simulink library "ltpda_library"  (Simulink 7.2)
settings: Solver=ode45  SolverMode=SingleTasking  StartTime=0.0  StopTime=10.0  RelTol=1e-3
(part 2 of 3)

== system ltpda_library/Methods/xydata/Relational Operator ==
  eq : Subsystem  Tag=method xydata  AncestorBlock=libraryBase/function
  ne : Subsystem  Tag=method xydata  AncestorBlock=libraryBase/function

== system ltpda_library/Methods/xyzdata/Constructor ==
  xyzdata : Subsystem  Tag=method xyzdata  AncestorBlock=libraryBase/constructor

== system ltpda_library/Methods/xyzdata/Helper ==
  isprop : Subsystem  Tag=method xyzdata  AncestorBlock=libraryBase/function

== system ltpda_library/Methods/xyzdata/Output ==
  char : Subsystem  Tag=method xyzdata  AncestorBlock=libraryBase/output
  display : Subsystem  Tag=method xyzdata  AncestorBlock=libraryBase/output

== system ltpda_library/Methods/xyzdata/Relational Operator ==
  eq : Subsystem  Tag=method xyzdata  AncestorBlock=libraryBase/function
  ne : Subsystem  Tag=method xyzdata  AncestorBlock=libraryBase/function

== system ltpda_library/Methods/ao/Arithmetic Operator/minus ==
  In1 : Inport  OutDataType=sfix(16)  OutScaling=2^0
  minus : M-S-Function  Tag=minus  FunctionName=ltpdasim
  Out1 : Outport  OutDataType=sfix(16)  OutScaling=2^0
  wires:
  In1/1 -> minus/1
  minus/1 -> Out1/1

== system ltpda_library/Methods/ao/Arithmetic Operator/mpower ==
  In1 : Inport  OutDataType=sfix(16)  OutScaling=2^0
  mpower : M-S-Function  Tag=mpower  FunctionName=ltpdasim
  Out1 : Outport  OutDataType=sfix(16)  OutScaling=2^0
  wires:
  In1/1 -> mpower/1
  mpower/1 -> Out1/1

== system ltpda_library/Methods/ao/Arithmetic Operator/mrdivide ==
  In1 : Inport  OutDataType=sfix(16)  OutScaling=2^0
  mrdivide : M-S-Function  Tag=mrdivide  FunctionName=ltpdasim
  Out1 : Outport  OutDataType=sfix(16)  OutScaling=2^0
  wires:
  In1/1 -> mrdivide/1
  mrdivide/1 -> Out1/1

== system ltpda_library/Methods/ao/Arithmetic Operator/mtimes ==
  In1 : Inport  OutDataType=sfix(16)  OutScaling=2^0
  mtimes : M-S-Function  Tag=mtimes  FunctionName=ltpdasim
  Out1 : Outport  OutDataType=sfix(16)  OutScaling=2^0
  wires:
  In1/1 -> mtimes/1
  mtimes/1 -> Out1/1

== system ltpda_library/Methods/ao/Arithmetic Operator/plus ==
  In1 : Inport  OutDataType=sfix(16)  OutScaling=2^0
  plus : M-S-Function  Tag=plus  FunctionName=ltpdasim
  Out1 : Outport  OutDataType=sfix(16)  OutScaling=2^0
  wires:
  In1/1 -> plus/1
  plus/1 -> Out1/1

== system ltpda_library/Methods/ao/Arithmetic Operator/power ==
  In1 : Inport  OutDataType=sfix(16)  OutScaling=2^0
  power : M-S-Function  Tag=power  FunctionName=ltpdasim
  Out1 : Outport  OutDataType=sfix(16)  OutScaling=2^0
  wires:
  In1/1 -> power/1
  power/1 -> Out1/1

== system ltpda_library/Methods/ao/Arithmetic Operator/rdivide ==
  In1 : Inport  OutDataType=sfix(16)  OutScaling=2^0
  rdivide : M-S-Function  Tag=rdivide  FunctionName=ltpdasim
  Out1 : Outport  OutDataType=sfix(16)  OutScaling=2^0
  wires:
  In1/1 -> rdivide/1
  rdivide/1 -> Out1/1

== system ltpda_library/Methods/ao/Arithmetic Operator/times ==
  In1 : Inport  OutDataType=sfix(16)  OutScaling=2^0
  times : M-S-Function  Tag=times  FunctionName=ltpdasim
  Out1 : Outport  OutDataType=sfix(16)  OutScaling=2^0
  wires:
  In1/1 -> times/1
  times/1 -> Out1/1

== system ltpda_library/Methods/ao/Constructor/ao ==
  Ground : Ground
  ao : M-S-Function  Tag=ao  FunctionName=ltpdasim
  Out1 : Outport  OutDataType=sfix(16)  OutScaling=2^0
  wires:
  Ground/1 -> ao/1
  ao/1 -> Out1/1

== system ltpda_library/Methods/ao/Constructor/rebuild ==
  Ground : Ground
  rebuild : M-S-Function  Tag=rebuild  FunctionName=ltpdasim
  Out1 : Outport  OutDataType=sfix(16)  OutScaling=2^0
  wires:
  Ground/1 -> rebuild/1
  rebuild/1 -> Out1/1

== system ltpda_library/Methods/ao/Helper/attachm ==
  In1 : Inport  OutDataType=sfix(16)  OutScaling=2^0
  attachm : M-S-Function  Tag=attachm  FunctionName=ltpdasim
  Out1 : Outport  OutDataType=sfix(16)  OutScaling=2^0
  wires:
  In1/1 -> attachm/1
  attachm/1 -> Out1/1

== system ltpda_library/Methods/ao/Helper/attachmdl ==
  In1 : Inport  OutDataType=sfix(16)  OutScaling=2^0
  attachmdl : M-S-Function  Tag=attachmdl  FunctionName=ltpdasim
  Out1 : Outport  OutDataType=sfix(16)  OutScaling=2^0
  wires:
  In1/1 -> attachmdl/1
  attachmdl/1 -> Out1/1

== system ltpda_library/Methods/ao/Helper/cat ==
  In1 : Inport  OutDataType=sfix(16)  OutScaling=2^0
  cat : M-S-Function  Tag=cat  FunctionName=ltpdasim
  Out1 : Outport  OutDataType=sfix(16)  OutScaling=2^0
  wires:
  In1/1 -> cat/1
  cat/1 -> Out1/1

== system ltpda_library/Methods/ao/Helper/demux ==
  In1 : Inport  OutDataType=sfix(16)  OutScaling=2^0
  demux : M-S-Function  Tag=demux  FunctionName=ltpdasim
  Out1 : Outport  OutDataType=sfix(16)  OutScaling=2^0
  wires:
  In1/1 -> demux/1
  demux/1 -> Out1/1

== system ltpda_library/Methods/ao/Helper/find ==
  In1 : Inport  OutDataType=sfix(16)  OutScaling=2^0
  find : M-S-Function  Tag=find  FunctionName=ltpdasim
  Out1 : Outport  OutDataType=sfix(16)  OutScaling=2^0
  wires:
  In1/1 -> find/1
  find/1 -> Out1/1

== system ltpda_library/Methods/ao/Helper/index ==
  In1 : Inport  OutDataType=sfix(16)  OutScaling=2^0
  index : M-S-Function  Tag=index  FunctionName=ltpdasim
  Out1 : Outport  OutDataType=sfix(16)  OutScaling=2^0
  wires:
  In1/1 -> index/1
  index/1 -> Out1/1

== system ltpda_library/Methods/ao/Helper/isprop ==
  In1 : Inport  OutDataType=sfix(16)  OutScaling=2^0
  isprop : M-S-Function  Tag=isprop  FunctionName=ltpdasim
  Out1 : Outport  OutDataType=sfix(16)  OutScaling=2^0
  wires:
  In1/1 -> isprop/1
  isprop/1 -> Out1/1

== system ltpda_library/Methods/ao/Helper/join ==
  In1 : Inport  OutDataType=sfix(16)  OutScaling=2^0
  join : M-S-Function  Tag=join  FunctionName=ltpdasim
  Out1 : Outport  OutDataType=sfix(16)  OutScaling=2^0
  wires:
  In1/1 -> join/1
  join/1 -> Out1/1

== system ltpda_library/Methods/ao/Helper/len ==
  In1 : Inport  OutDataType=sfix(16)  OutScaling=2^0
  len : M-S-Function  Tag=len  FunctionName=ltpdasim
  Out1 : Outport  OutDataType=sfix(16)  OutScaling=2^0
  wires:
  In1/1 -> len/1
  len/1 -> Out1/1

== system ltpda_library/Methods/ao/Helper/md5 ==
  In1 : Inport  OutDataType=sfix(16)  OutScaling=2^0
  md5 : M-S-Function  Tag=md5  FunctionName=ltpdasim
  Out1 : Outport  OutDataType=sfix(16)  OutScaling=2^0
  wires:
  In1/1 -> md5/1
  md5/1 -> Out1/1

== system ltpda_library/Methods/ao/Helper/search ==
  In1 : Inport  OutDataType=sfix(16)  OutScaling=2^0
  search : M-S-Function  Tag=search  FunctionName=ltpdasim
  Out1 : Outport  OutDataType=sfix(16)  OutScaling=2^0
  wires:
  In1/1 -> search/1
  search/1 -> Out1/1

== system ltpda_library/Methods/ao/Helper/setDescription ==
  In1 : Inport  OutDataType=sfix(16)  OutScaling=2^0
  setDescription : M-S-Function  Tag=setDescription  FunctionName=ltpdasim
  Out1 : Outport  OutDataType=sfix(16)  OutScaling=2^0
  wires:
  In1/1 -> setDescription/1
  setDescription/1 -> Out1/1

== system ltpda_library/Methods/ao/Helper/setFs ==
  In1 : Inport  OutDataType=sfix(16)  OutScaling=2^0
  setFs : M-S-Function  Tag=setFs  FunctionName=ltpdasim
  Out1 : Outport  OutDataType=sfix(16)  OutScaling=2^0
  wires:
  In1/1 -> setFs/1
  setFs/1 -> Out1/1

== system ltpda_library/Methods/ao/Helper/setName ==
  In1 : Inport  OutDataType=sfix(16)  OutScaling=2^0
  setName : M-S-Function  Tag=setName  FunctionName=ltpdasim
  Out1 : Outport  OutDataType=sfix(16)  OutScaling=2^0
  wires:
  In1/1 -> setName/1
  setName/1 -> Out1/1

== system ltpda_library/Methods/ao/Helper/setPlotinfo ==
  In1 : Inport  OutDataType=sfix(16)  OutScaling=2^0
  setPlotinfo : M-S-Function  Tag=setPlotinfo  FunctionName=ltpdasim
  Out1 : Outport  OutDataType=sfix(16)  OutScaling=2^0
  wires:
  In1/1 -> setPlotinfo/1
  setPlotinfo/1 -> Out1/1

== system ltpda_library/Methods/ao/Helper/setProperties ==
  In1 : Inport  OutDataType=sfix(16)  OutScaling=2^0
  setProperties : M-S-Function  Tag=setProperties  FunctionName=ltpdasim
  Out1 : Outport  OutDataType=sfix(16)  OutScaling=2^0
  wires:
  In1/1 -> setProperties/1
  setProperties/1 -> Out1/1

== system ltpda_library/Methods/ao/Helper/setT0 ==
  In1 : Inport  OutDataType=sfix(16)  OutScaling=2^0
  setT0 : M-S-Function  Tag=setT0  FunctionName=ltpdasim
  Out1 : Outport  OutDataType=sfix(16)  OutScaling=2^0
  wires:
  In1/1 -> setT0/1
  setT0/1 -> Out1/1

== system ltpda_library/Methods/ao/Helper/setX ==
  In1 : Inport  OutDataType=sfix(16)  OutScaling=2^0
  setX : M-S-Function  Tag=setX  FunctionName=ltpdasim
  Out1 : Outport  OutDataType=sfix(16)  OutScaling=2^0
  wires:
  In1/1 -> setX/1
  setX/1 -> Out1/1

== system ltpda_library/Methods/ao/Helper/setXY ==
  In1 : Inport  OutDataType=sfix(16)  OutScaling=2^0
  setXY : M-S-Function  Tag=setXY  FunctionName=ltpdasim
  Out1 : Outport  OutDataType=sfix(16)  OutScaling=2^0
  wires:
  In1/1 -> setXY/1
  setXY/1 -> Out1/1

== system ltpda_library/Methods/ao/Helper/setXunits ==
  In1 : Inport  OutDataType=sfix(16)  OutScaling=2^0
  setXunits : M-S-Function  Tag=setXunits  FunctionName=ltpdasim
  Out1 : Outport  OutDataType=sfix(16)  OutScaling=2^0
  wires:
  In1/1 -> setXunits/1
  setXunits/1 -> Out1/1

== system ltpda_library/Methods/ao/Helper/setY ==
  In1 : Inport  OutDataType=sfix(16)  OutScaling=2^0
  setY : M-S-Function  Tag=setY  FunctionName=ltpdasim
  Out1 : Outport  OutDataType=sfix(16)  OutScaling=2^0
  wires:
  In1/1 -> setY/1
  setY/1 -> Out1/1

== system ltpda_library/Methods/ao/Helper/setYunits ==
  In1 : Inport  OutDataType=sfix(16)  OutScaling=2^0
  setYunits : M-S-Function  Tag=setYunits  FunctionName=ltpdasim
  Out1 : Outport  OutDataType=sfix(16)  OutScaling=2^0
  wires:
  In1/1 -> setYunits/1
  setYunits/1 -> Out1/1

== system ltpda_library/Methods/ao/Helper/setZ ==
  In1 : Inport  OutDataType=sfix(16)  OutScaling=2^0
  setZ : M-S-Function  Tag=setZ  FunctionName=ltpdasim
  Out1 : Outport  OutDataType=sfix(16)  OutScaling=2^0
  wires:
  In1/1 -> setZ/1
  setZ/1 -> Out1/1

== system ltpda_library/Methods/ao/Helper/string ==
  In1 : Inport  OutDataType=sfix(16)  OutScaling=2^0
  string : M-S-Function  Tag=string  FunctionName=ltpdasim
  Out1 : Outport  OutDataType=sfix(16)  OutScaling=2^0
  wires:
  In1/1 -> string/1
  string/1 -> Out1/1

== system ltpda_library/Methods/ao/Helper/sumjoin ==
  In1 : Inport  OutDataType=sfix(16)  OutScaling=2^0
  sumjoin : M-S-Function  Tag=sumjoin  FunctionName=ltpdasim
  Out1 : Outport  OutDataType=sfix(16)  OutScaling=2^0
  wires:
  In1/1 -> sumjoin/1
  sumjoin/1 -> Out1/1

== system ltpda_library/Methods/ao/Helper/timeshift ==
  In1 : Inport  OutDataType=sfix(16)  OutScaling=2^0
  timeshift : M-S-Function  Tag=timeshift  FunctionName=ltpdasim
  Out1 : Outport  OutDataType=sfix(16)  OutScaling=2^0
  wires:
  In1/1 -> timeshift/1
  timeshift/1 -> Out1/1

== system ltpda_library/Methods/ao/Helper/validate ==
  In1 : Inport  OutDataType=sfix(16)  OutScaling=2^0
  validate : M-S-Function  Tag=validate  FunctionName=ltpdasim
  Out1 : Outport  OutDataType=sfix(16)  OutScaling=2^0
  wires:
  In1/1 -> validate/1
  validate/1 -> Out1/1

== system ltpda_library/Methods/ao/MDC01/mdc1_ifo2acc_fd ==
  In1 : Inport  OutDataType=sfix(16)  OutScaling=2^0
  mdc1_ifo2acc_fd : M-S-Function  Tag=mdc1_ifo2acc_fd  FunctionName=ltpdasim
  Out1 : Outport  OutDataType=sfix(16)  OutScaling=2^0
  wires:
  In1/1 -> mdc1_ifo2acc_fd/1
  mdc1_ifo2acc_fd/1 -> Out1/1

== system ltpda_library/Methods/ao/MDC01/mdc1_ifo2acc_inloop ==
  In1 : Inport  OutDataType=sfix(16)  OutScaling=2^0
  mdc1_ifo2acc_inloop : M-S-Function  Tag=mdc1_ifo2acc_inloop  FunctionName=ltpdasim
  Out1 : Outport  OutDataType=sfix(16)  OutScaling=2^0
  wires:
  In1/1 -> mdc1_ifo2acc_inloop/1
  mdc1_ifo2acc_inloop/1 -> Out1/1

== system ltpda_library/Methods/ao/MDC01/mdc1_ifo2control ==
  In1 : Inport  OutDataType=sfix(16)  OutScaling=2^0
  mdc1_ifo2control : M-S-Function  Tag=mdc1_ifo2control  FunctionName=ltpdasim
  Out1 : Outport  OutDataType=sfix(16)  OutScaling=2^0
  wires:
  In1/1 -> mdc1_ifo2control/1
  mdc1_ifo2control/1 -> Out1/1

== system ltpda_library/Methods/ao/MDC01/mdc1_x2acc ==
  In1 : Inport  OutDataType=sfix(16)  OutScaling=2^0
  mdc1_x2acc : M-S-Function  Tag=mdc1_x2acc  FunctionName=ltpdasim
  Out1 : Outport  OutDataType=sfix(16)  OutScaling=2^0
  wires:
  In1/1 -> mdc1_x2acc/1
  mdc1_x2acc/1 -> Out1/1

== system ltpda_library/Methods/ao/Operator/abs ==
  In1 : Inport  OutDataType=sfix(16)  OutScaling=2^0
  abs : M-S-Function  Tag=abs  FunctionName=ltpdasim
  Out1 : Outport  OutDataType=sfix(16)  OutScaling=2^0
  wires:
  In1/1 -> abs/1
  abs/1 -> Out1/1

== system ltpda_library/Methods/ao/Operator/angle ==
  In1 : Inport  OutDataType=sfix(16)  OutScaling=2^0
  angle : M-S-Function  Tag=angle  FunctionName=ltpdasim
  Out1 : Outport  OutDataType=sfix(16)  OutScaling=2^0
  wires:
  In1/1 -> angle/1
  angle/1 -> Out1/1

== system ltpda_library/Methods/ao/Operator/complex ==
  In1 : Inport  OutDataType=sfix(16)  OutScaling=2^0
  complex : M-S-Function  Tag=complex  FunctionName=ltpdasim
  Out1 : Outport  OutDataType=sfix(16)  OutScaling=2^0
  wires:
  In1/1 -> complex/1
  complex/1 -> Out1/1

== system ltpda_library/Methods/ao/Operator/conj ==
  In1 : Inport  OutDataType=sfix(16)  OutScaling=2^0
  conj : M-S-Function  Tag=conj  FunctionName=ltpdasim
  Out1 : Outport  OutDataType=sfix(16)  OutScaling=2^0
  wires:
  In1/1 -> conj/1
  conj/1 -> Out1/1

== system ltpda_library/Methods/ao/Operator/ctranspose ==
  In1 : Inport  OutDataType=sfix(16)  OutScaling=2^0
  ctranspose : M-S-Function  Tag=ctranspose  FunctionName=ltpdasim
  Out1 : Outport  OutDataType=sfix(16)  OutScaling=2^0
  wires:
  In1/1 -> ctranspose/1
  ctranspose/1 -> Out1/1

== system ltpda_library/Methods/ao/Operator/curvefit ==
  In1 : Inport  OutDataType=sfix(16)  OutScaling=2^0
  curvefit : M-S-Function  Tag=curvefit  FunctionName=ltpdasim
  Out1 : Outport  OutDataType=sfix(16)  OutScaling=2^0
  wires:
  In1/1 -> curvefit/1
  curvefit/1 -> Out1/1

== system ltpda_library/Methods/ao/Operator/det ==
  In1 : Inport  OutDataType=sfix(16)  OutScaling=2^0
  det : M-S-Function  Tag=det  FunctionName=ltpdasim
  Out1 : Outport  OutDataType=sfix(16)  OutScaling=2^0
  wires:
  In1/1 -> det/1
  det/1 -> Out1/1

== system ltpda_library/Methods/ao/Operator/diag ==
  In1 : Inport  OutDataType=sfix(16)  OutScaling=2^0
  diag : M-S-Function  Tag=diag  FunctionName=ltpdasim
  Out1 : Outport  OutDataType=sfix(16)  OutScaling=2^0
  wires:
  In1/1 -> diag/1
  diag/1 -> Out1/1

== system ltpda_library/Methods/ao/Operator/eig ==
  In1 : Inport  OutDataType=sfix(16)  OutScaling=2^0
  eig : M-S-Function  Tag=eig  FunctionName=ltpdasim
  Out1 : Outport  OutDataType=sfix(16)  OutScaling=2^0
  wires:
  In1/1 -> eig/1
  eig/1 -> Out1/1

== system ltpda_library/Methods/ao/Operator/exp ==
  In1 : Inport  OutDataType=sfix(16)  OutScaling=2^0
  exp : M-S-Function  Tag=exp  FunctionName=ltpdasim
  Out1 : Outport  OutDataType=sfix(16)  OutScaling=2^0
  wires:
  In1/1 -> exp/1
  exp/1 -> Out1/1

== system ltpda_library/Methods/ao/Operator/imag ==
  In1 : Inport  OutDataType=sfix(16)  OutScaling=2^0
  imag : M-S-Function  Tag=imag  FunctionName=ltpdasim
  Out1 : Outport  OutDataType=sfix(16)  OutScaling=2^0
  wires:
  In1/1 -> imag/1
  imag/1 -> Out1/1

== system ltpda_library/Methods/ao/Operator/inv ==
  In1 : Inport  OutDataType=sfix(16)  OutScaling=2^0
  inv : M-S-Function  Tag=inv  FunctionName=ltpdasim
  Out1 : Outport  OutDataType=sfix(16)  OutScaling=2^0
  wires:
  In1/1 -> inv/1
  inv/1 -> Out1/1

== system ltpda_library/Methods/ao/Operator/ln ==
  In1 : Inport  OutDataType=sfix(16)  OutScaling=2^0
  ln : M-S-Function  Tag=ln  FunctionName=ltpdasim
  Out1 : Outport  OutDataType=sfix(16)  OutScaling=2^0
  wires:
  In1/1 -> ln/1
  ln/1 -> Out1/1

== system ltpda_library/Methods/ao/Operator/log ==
  In1 : Inport  OutDataType=sfix(16)  OutScaling=2^0
  log : M-S-Function  Tag=log  FunctionName=ltpdasim
  Out1 : Outport  OutDataType=sfix(16)  OutScaling=2^0
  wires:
  In1/1 -> log/1
  log/1 -> Out1/1

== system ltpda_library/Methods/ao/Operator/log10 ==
  In1 : Inport  OutDataType=sfix(16)  OutScaling=2^0
  log10 : M-S-Function  Tag=log10  FunctionName=ltpdasim
  Out1 : Outport  OutDataType=sfix(16)  OutScaling=2^0
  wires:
  In1/1 -> log10/1
  log10/1 -> Out1/1

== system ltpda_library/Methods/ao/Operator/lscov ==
  In1 : Inport  OutDataType=sfix(16)  OutScaling=2^0
  lscov : M-S-Function  Tag=lscov  FunctionName=ltpdasim
  Out1 : Outport  OutDataType=sfix(16)  OutScaling=2^0
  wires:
  In1/1 -> lscov/1
  lscov/1 -> Out1/1

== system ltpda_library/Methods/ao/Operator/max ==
  In1 : Inport  OutDataType=sfix(16)  OutScaling=2^0
  max : M-S-Function  Tag=max  FunctionName=ltpdasim
  Out1 : Outport  OutDataType=sfix(16)  OutScaling=2^0
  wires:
  In1/1 -> max/1
  max/1 -> Out1/1

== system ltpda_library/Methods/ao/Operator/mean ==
  In1 : Inport  OutDataType=sfix(16)  OutScaling=2^0
  mean : M-S-Function  Tag=mean  FunctionName=ltpdasim
  Out1 : Outport  OutDataType=sfix(16)  OutScaling=2^0
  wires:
  In1/1 -> mean/1
  mean/1 -> Out1/1

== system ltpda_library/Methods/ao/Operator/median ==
  In1 : Inport  OutDataType=sfix(16)  OutScaling=2^0
  median : M-S-Function  Tag=median  FunctionName=ltpdasim
  Out1 : Outport  OutDataType=sfix(16)  OutScaling=2^0
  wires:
  In1/1 -> median/1
  median/1 -> Out1/1

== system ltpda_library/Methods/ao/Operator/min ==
  In1 : Inport  OutDataType=sfix(16)  OutScaling=2^0
  min : M-S-Function  Tag=min  FunctionName=ltpdasim
  Out1 : Outport  OutDataType=sfix(16)  OutScaling=2^0
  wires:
  In1/1 -> min/1
  min/1 -> Out1/1

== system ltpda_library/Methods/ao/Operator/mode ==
  In1 : Inport  OutDataType=sfix(16)  OutScaling=2^0
  mode : M-S-Function  Tag=mode  FunctionName=ltpdasim
  Out1 : Outport  OutDataType=sfix(16)  OutScaling=2^0
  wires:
  In1/1 -> mode/1
  mode/1 -> Out1/1

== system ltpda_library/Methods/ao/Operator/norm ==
  In1 : Inport  OutDataType=sfix(16)  OutScaling=2^0
  norm : M-S-Function  Tag=norm  FunctionName=ltpdasim
  Out1 : Outport  OutDataType=sfix(16)  OutScaling=2^0
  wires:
  In1/1 -> norm/1
  norm/1 -> Out1/1

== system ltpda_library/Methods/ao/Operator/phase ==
  In1 : Inport  OutDataType=sfix(16)  OutScaling=2^0
  phase : M-S-Function  Tag=phase  FunctionName=ltpdasim
  Out1 : Outport  OutDataType=sfix(16)  OutScaling=2^0
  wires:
  In1/1 -> phase/1
  phase/1 -> Out1/1

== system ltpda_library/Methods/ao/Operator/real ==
  In1 : Inport  OutDataType=sfix(16)  OutScaling=2^0
  real : M-S-Function  Tag=real  FunctionName=ltpdasim
  Out1 : Outport  OutDataType=sfix(16)  OutScaling=2^0
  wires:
  In1/1 -> real/1
  real/1 -> Out1/1

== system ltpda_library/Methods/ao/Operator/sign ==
  In1 : Inport  OutDataType=sfix(16)  OutScaling=2^0
  sign : M-S-Function  Tag=sign  FunctionName=ltpdasim
  Out1 : Outport  OutDataType=sfix(16)  OutScaling=2^0
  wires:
  In1/1 -> sign/1
  sign/1 -> Out1/1

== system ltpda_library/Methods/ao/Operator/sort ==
  In1 : Inport  OutDataType=sfix(16)  OutScaling=2^0
  sort : M-S-Function  Tag=sort  FunctionName=ltpdasim
  Out1 : Outport  OutDataType=sfix(16)  OutScaling=2^0
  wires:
  In1/1 -> sort/1
  sort/1 -> Out1/1

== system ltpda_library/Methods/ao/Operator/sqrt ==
  In1 : Inport  OutDataType=sfix(16)  OutScaling=2^0
  sqrt : M-S-Function  Tag=sqrt  FunctionName=ltpdasim
  Out1 : Outport  OutDataType=sfix(16)  OutScaling=2^0
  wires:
  In1/1 -> sqrt/1
  sqrt/1 -> Out1/1

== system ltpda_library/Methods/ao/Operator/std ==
  In1 : Inport  OutDataType=sfix(16)  OutScaling=2^0
  std : M-S-Function  Tag=std  FunctionName=ltpdasim
  Out1 : Outport  OutDataType=sfix(16)  OutScaling=2^0
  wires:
  In1/1 -> std/1
  std/1 -> Out1/1

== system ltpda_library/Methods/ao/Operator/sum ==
  In1 : Inport  OutDataType=sfix(16)  OutScaling=2^0
  sum : M-S-Function  Tag=sum  FunctionName=ltpdasim
  Out1 : Outport  OutDataType=sfix(16)  OutScaling=2^0
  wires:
  In1/1 -> sum/1
  sum/1 -> Out1/1

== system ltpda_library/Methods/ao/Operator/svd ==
  In1 : Inport  OutDataType=sfix(16)  OutScaling=2^0
  svd : M-S-Function  Tag=svd  FunctionName=ltpdasim
  Out1 : Outport  OutDataType=sfix(16)  OutScaling=2^0
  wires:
  In1/1 -> svd/1
  svd/1 -> Out1/1

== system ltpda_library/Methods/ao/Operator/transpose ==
  In1 : Inport  OutDataType=sfix(16)  OutScaling=2^0
  transpose : M-S-Function  Tag=transpose  FunctionName=ltpdasim
  Out1 : Outport  OutDataType=sfix(16)  OutScaling=2^0
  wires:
  In1/1 -> transpose/1
  transpose/1 -> Out1/1

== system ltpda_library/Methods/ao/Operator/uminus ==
  In1 : Inport  OutDataType=sfix(16)  OutScaling=2^0
  uminus : M-S-Function  Tag=uminus  FunctionName=ltpdasim
  Out1 : Outport  OutDataType=sfix(16)  OutScaling=2^0
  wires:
  In1/1 -> uminus/1
  uminus/1 -> Out1/1

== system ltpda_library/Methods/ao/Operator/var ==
  In1 : Inport  OutDataType=sfix(16)  OutScaling=2^0
  var : M-S-Function  Tag=var  FunctionName=ltpdasim
  Out1 : Outport  OutDataType=sfix(16)  OutScaling=2^0
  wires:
  In1/1 -> var/1
  var/1 -> Out1/1

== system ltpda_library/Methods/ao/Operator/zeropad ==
  In1 : Inport  OutDataType=sfix(16)  OutScaling=2^0
  zeropad : M-S-Function  Tag=zeropad  FunctionName=ltpdasim
  Out1 : Outport  OutDataType=sfix(16)  OutScaling=2^0
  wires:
  In1/1 -> zeropad/1
  zeropad/1 -> Out1/1

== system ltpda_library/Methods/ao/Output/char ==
  In1 : Inport  OutDataType=sfix(16)  OutScaling=2^0
  Terminator : Terminator
  char : M-S-Function  Tag=char  FunctionName=ltpdasim
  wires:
  char/1 -> Terminator/1
  In1/1 -> char/1

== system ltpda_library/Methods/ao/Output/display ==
  In1 : Inport  OutDataType=sfix(16)  OutScaling=2^0
  Terminator : Terminator
  display : M-S-Function  Tag=display  FunctionName=ltpdasim
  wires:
  display/1 -> Terminator/1
  In1/1 -> display/1

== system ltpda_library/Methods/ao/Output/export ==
  In1 : Inport  OutDataType=sfix(16)  OutScaling=2^0
  Terminator : Terminator
  export : M-S-Function  Tag=export  FunctionName=ltpdasim
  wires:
  export/1 -> Terminator/1
  In1/1 -> export/1

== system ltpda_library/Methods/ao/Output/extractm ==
  In1 : Inport  OutDataType=sfix(16)  OutScaling=2^0
  Terminator : Terminator
  extractm : M-S-Function  Tag=extractm  FunctionName=ltpdasim
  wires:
  extractm/1 -> Terminator/1
  In1/1 -> extractm/1

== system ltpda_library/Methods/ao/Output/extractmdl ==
  In1 : Inport  OutDataType=sfix(16)  OutScaling=2^0
  Terminator : Terminator
  extractmdl : M-S-Function  Tag=extractmdl  FunctionName=ltpdasim
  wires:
  extractmdl/1 -> Terminator/1
  In1/1 -> extractmdl/1

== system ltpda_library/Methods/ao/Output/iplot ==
  In1 : Inport  OutDataType=sfix(16)  OutScaling=2^0
  Terminator : Terminator
  iplot : M-S-Function  Tag=iplot  FunctionName=ltpdasim
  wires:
  iplot/1 -> Terminator/1
  In1/1 -> iplot/1

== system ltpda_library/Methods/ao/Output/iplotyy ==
  In1 : Inport  OutDataType=sfix(16)  OutScaling=2^0
  Terminator : Terminator
  iplotyy : M-S-Function  Tag=iplotyy  FunctionName=ltpdasim
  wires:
  iplotyy/1 -> Terminator/1
  In1/1 -> iplotyy/1

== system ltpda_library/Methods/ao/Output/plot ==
  In1 : Inport  OutDataType=sfix(16)  OutScaling=2^0
  Terminator : Terminator
  plot : M-S-Function  Tag=plot  FunctionName=ltpdasim
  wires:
  plot/1 -> Terminator/1
  In1/1 -> plot/1

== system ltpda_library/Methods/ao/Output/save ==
  In1 : Inport  OutDataType=sfix(16)  OutScaling=2^0
  Terminator : Terminator
  save : M-S-Function  Tag=save  FunctionName=ltpdasim
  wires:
  save/1 -> Terminator/1
  In1/1 -> save/1

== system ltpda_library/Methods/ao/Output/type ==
  In1 : Inport  OutDataType=sfix(16)  OutScaling=2^0
  Terminator : Terminator
  type : M-S-Function  Tag=type  FunctionName=ltpdasim
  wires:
  type/1 -> Terminator/1
  In1/1 -> type/1

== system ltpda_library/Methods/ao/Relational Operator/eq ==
  In1 : Inport  OutDataType=sfix(16)  OutScaling=2^0
  eq : M-S-Function  Tag=eq  FunctionName=ltpdasim
  Out1 : Outport  OutDataType=sfix(16)  OutScaling=2^0
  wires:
  In1/1 -> eq/1
  eq/1 -> Out1/1

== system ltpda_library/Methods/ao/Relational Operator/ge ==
  In1 : Inport  OutDataType=sfix(16)  OutScaling=2^0
  ge : M-S-Function  Tag=ge  FunctionName=ltpdasim
  Out1 : Outport  OutDataType=sfix(16)  OutScaling=2^0
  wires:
  In1/1 -> ge/1
  ge/1 -> Out1/1

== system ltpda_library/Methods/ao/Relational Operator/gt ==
  In1 : Inport  OutDataType=sfix(16)  OutScaling=2^0
  gt : M-S-Function  Tag=gt  FunctionName=ltpdasim
  Out1 : Outport  OutDataType=sfix(16)  OutScaling=2^0
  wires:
  In1/1 -> gt/1
  gt/1 -> Out1/1

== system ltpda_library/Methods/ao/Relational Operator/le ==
  In1 : Inport  OutDataType=sfix(16)  OutScaling=2^0
  le : M-S-Function  Tag=le  FunctionName=ltpdasim
  Out1 : Outport  OutDataType=sfix(16)  OutScaling=2^0
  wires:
  In1/1 -> le/1
  le/1 -> Out1/1

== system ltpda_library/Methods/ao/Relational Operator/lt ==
  In1 : Inport  OutDataType=sfix(16)  OutScaling=2^0
  lt : M-S-Function  Tag=lt  FunctionName=ltpdasim
  Out1 : Outport  OutDataType=sfix(16)  OutScaling=2^0
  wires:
  In1/1 -> lt/1
  lt/1 -> Out1/1

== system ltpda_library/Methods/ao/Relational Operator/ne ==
  In1 : Inport  OutDataType=sfix(16)  OutScaling=2^0
  ne : M-S-Function  Tag=ne  FunctionName=ltpdasim
  Out1 : Outport  OutDataType=sfix(16)  OutScaling=2^0
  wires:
  In1/1 -> ne/1
  ne/1 -> Out1/1

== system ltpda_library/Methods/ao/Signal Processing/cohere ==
  In1 : Inport  OutDataType=sfix(16)  OutScaling=2^0
  cohere : M-S-Function  Tag=cohere  FunctionName=ltpdasim
  Out1 : Outport  OutDataType=sfix(16)  OutScaling=2^0
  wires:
  In1/1 -> cohere/1
  cohere/1 -> Out1/1

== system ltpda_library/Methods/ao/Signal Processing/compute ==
  In1 : Inport  OutDataType=sfix(16)  OutScaling=2^0
  compute : M-S-Function  Tag=compute  FunctionName=ltpdasim
  Out1 : Outport  OutDataType=sfix(16)  OutScaling=2^0
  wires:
  In1/1 -> compute/1
  compute/1 -> Out1/1

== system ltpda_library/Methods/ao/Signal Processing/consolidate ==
  In1 : Inport  OutDataType=sfix(16)  OutScaling=2^0
  consolidate : M-S-Function  Tag=consolidate  FunctionName=ltpdasim
  Out1 : Outport  OutDataType=sfix(16)  OutScaling=2^0
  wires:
  In1/1 -> consolidate/1
  consolidate/1 -> Out1/1

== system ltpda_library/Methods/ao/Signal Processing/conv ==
  In1 : Inport  OutDataType=sfix(16)  OutScaling=2^0
  conv : M-S-Function  Tag=conv  FunctionName=ltpdasim
  Out1 : Outport  OutDataType=sfix(16)  OutScaling=2^0
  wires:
  In1/1 -> conv/1
  conv/1 -> Out1/1

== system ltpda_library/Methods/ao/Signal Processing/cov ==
  In1 : Inport  OutDataType=sfix(16)  OutScaling=2^0
  cov : M-S-Function  Tag=cov  FunctionName=ltpdasim
  Out1 : Outport  OutDataType=sfix(16)  OutScaling=2^0
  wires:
  In1/1 -> cov/1
  cov/1 -> Out1/1

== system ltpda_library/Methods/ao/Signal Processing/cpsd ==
  In1 : Inport  OutDataType=sfix(16)  OutScaling=2^0
  cpsd : M-S-Function  Tag=cpsd  FunctionName=ltpdasim
  Out1 : Outport  OutDataType=sfix(16)  OutScaling=2^0
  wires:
  In1/1 -> cpsd/1
  cpsd/1 -> Out1/1

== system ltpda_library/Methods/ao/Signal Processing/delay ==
  In1 : Inport  OutDataType=sfix(16)  OutScaling=2^0
  delay : M-S-Function  Tag=delay  FunctionName=ltpdasim
  Out1 : Outport  OutDataType=sfix(16)  OutScaling=2^0
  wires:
  In1/1 -> delay/1
  delay/1 -> Out1/1

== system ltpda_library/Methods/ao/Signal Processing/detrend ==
  In1 : Inport  OutDataType=sfix(16)  OutScaling=2^0
  detrend : M-S-Function  Tag=detrend  FunctionName=ltpdasim
  Out1 : Outport  OutDataType=sfix(16)  OutScaling=2^0
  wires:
  In1/1 -> detrend/1
  detrend/1 -> Out1/1

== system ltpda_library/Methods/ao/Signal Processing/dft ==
  In1 : Inport  OutDataType=sfix(16)  OutScaling=2^0
  dft : M-S-Function  Tag=dft  FunctionName=ltpdasim
  Out1 : Outport  OutDataType=sfix(16)  OutScaling=2^0
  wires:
  In1/1 -> dft/1
  dft/1 -> Out1/1

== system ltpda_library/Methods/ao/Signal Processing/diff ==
  In1 : Inport  OutDataType=sfix(16)  OutScaling=2^0
  diff : M-S-Function  Tag=diff  FunctionName=ltpdasim
  Out1 : Outport  OutDataType=sfix(16)  OutScaling=2^0
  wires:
  In1/1 -> diff/1
  diff/1 -> Out1/1

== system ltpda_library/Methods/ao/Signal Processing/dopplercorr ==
  In1 : Inport  OutDataType=sfix(16)  OutScaling=2^0
  dopplercorr : M-S-Function  Tag=dopplercorr  FunctionName=ltpdasim
  Out1 : Outport  OutDataType=sfix(16)  OutScaling=2^0
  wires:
  In1/1 -> dopplercorr/1
  dopplercorr/1 -> Out1/1

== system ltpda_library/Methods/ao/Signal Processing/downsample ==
  In1 : Inport  OutDataType=sfix(16)  OutScaling=2^0
  downsample : M-S-Function  Tag=downsample  FunctionName=ltpdasim
  Out1 : Outport  OutDataType=sfix(16)  OutScaling=2^0
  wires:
  In1/1 -> downsample/1
  downsample/1 -> Out1/1

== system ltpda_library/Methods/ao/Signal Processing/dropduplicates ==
  In1 : Inport  OutDataType=sfix(16)  OutScaling=2^0
  dropduplicates : M-S-Function  Tag=dropduplicates  FunctionName=ltpdasim
  Out1 : Outport  OutDataType=sfix(16)  OutScaling=2^0
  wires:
  In1/1 -> dropduplicates/1
  dropduplicates/1 -> Out1/1

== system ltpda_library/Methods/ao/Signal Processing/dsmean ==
  In1 : Inport  OutDataType=sfix(16)  OutScaling=2^0
  dsmean : M-S-Function  Tag=dsmean  FunctionName=ltpdasim
  Out1 : Outport  OutDataType=sfix(16)  OutScaling=2^0
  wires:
  In1/1 -> dsmean/1
  dsmean/1 -> Out1/1

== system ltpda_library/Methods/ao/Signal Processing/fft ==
  In1 : Inport  OutDataType=sfix(16)  OutScaling=2^0
  fft : M-S-Function  Tag=fft  FunctionName=ltpdasim
  Out1 : Outport  OutDataType=sfix(16)  OutScaling=2^0
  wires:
  In1/1 -> fft/1
  fft/1 -> Out1/1

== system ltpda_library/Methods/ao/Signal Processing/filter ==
  In1 : Inport  OutDataType=sfix(16)  OutScaling=2^0
  filter : M-S-Function  Tag=filter  FunctionName=ltpdasim
  Out1 : Outport  OutDataType=sfix(16)  OutScaling=2^0
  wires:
  In1/1 -> filter/1
  filter/1 -> Out1/1

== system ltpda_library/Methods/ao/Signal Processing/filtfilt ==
  In1 : Inport  OutDataType=sfix(16)  OutScaling=2^0
  filtfilt : M-S-Function  Tag=filtfilt  FunctionName=ltpdasim
  Out1 : Outport  OutDataType=sfix(16)  OutScaling=2^0
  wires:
  In1/1 -> filtfilt/1
  filtfilt/1 -> Out1/1

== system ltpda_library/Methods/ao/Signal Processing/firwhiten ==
  In1 : Inport  OutDataType=sfix(16)  OutScaling=2^0
  firwhiten : M-S-Function  Tag=firwhiten  FunctionName=ltpdasim
  Out1 : Outport  OutDataType=sfix(16)  OutScaling=2^0
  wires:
  In1/1 -> firwhiten/1
  firwhiten/1 -> Out1/1

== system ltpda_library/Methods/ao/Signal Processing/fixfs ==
  In1 : Inport  OutDataType=sfix(16)  OutScaling=2^0
  fixfs : M-S-Function  Tag=fixfs  FunctionName=ltpdasim
  Out1 : Outport  OutDataType=sfix(16)  OutScaling=2^0
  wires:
  In1/1 -> fixfs/1
  fixfs/1 -> Out1/1

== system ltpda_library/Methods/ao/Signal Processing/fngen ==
  In1 : Inport  OutDataType=sfix(16)  OutScaling=2^0
  fngen : M-S-Function  Tag=fngen  FunctionName=ltpdasim
  Out1 : Outport  OutDataType=sfix(16)  OutScaling=2^0
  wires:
  In1/1 -> fngen/1
  fngen/1 -> Out1/1

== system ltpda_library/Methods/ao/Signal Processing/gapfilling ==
  In1 : Inport  OutDataType=sfix(16)  OutScaling=2^0
  gapfilling : M-S-Function  Tag=gapfilling  FunctionName=ltpdasim
  Out1 : Outport  OutDataType=sfix(16)  OutScaling=2^0
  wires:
  In1/1 -> gapfilling/1
  gapfilling/1 -> Out1/1

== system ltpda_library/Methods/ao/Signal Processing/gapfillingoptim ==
  In1 : Inport  OutDataType=sfix(16)  OutScaling=2^0
  gapfillingoptim : M-S-Function  Tag=gapfillingoptim  FunctionName=ltpdasim
  Out1 : Outport  OutDataType=sfix(16)  OutScaling=2^0
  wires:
  In1/1 -> gapfillingoptim/1
  gapfillingoptim/1 -> Out1/1

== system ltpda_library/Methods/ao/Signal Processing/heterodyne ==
  In1 : Inport  OutDataType=sfix(16)  OutScaling=2^0
  heterodyne : M-S-Function  Tag=heterodyne  FunctionName=ltpdasim
  Out1 : Outport  OutDataType=sfix(16)  OutScaling=2^0
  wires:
  In1/1 -> heterodyne/1
  heterodyne/1 -> Out1/1

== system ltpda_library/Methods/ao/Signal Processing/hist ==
  In1 : Inport  OutDataType=sfix(16)  OutScaling=2^0
  hist : M-S-Function  Tag=hist  FunctionName=ltpdasim
  Out1 : Outport  OutDataType=sfix(16)  OutScaling=2^0
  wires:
  In1/1 -> hist/1
  hist/1 -> Out1/1

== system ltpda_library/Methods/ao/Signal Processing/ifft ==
  In1 : Inport  OutDataType=sfix(16)  OutScaling=2^0
  ifft : M-S-Function  Tag=ifft  FunctionName=ltpdasim
  Out1 : Outport  OutDataType=sfix(16)  OutScaling=2^0
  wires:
  In1/1 -> ifft/1
  ifft/1 -> Out1/1

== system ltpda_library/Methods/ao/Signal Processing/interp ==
  In1 : Inport  OutDataType=sfix(16)  OutScaling=2^0
  interp : M-S-Function  Tag=interp  FunctionName=ltpdasim
  Out1 : Outport  OutDataType=sfix(16)  OutScaling=2^0
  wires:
  In1/1 -> interp/1
  interp/1 -> Out1/1

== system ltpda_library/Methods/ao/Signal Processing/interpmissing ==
  In1 : Inport  OutDataType=sfix(16)  OutScaling=2^0
  interpmissing : M-S-Function  Tag=interpmissing  FunctionName=ltpdasim
  Out1 : Outport  OutDataType=sfix(16)  OutScaling=2^0
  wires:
  In1/1 -> interpmissing/1
  interpmissing/1 -> Out1/1

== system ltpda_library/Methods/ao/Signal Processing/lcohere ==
  In1 : Inport  OutDataType=sfix(16)  OutScaling=2^0
  lcohere : M-S-Function  Tag=lcohere  FunctionName=ltpdasim
  Out1 : Outport  OutDataType=sfix(16)  OutScaling=2^0
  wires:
  In1/1 -> lcohere/1
  lcohere/1 -> Out1/1

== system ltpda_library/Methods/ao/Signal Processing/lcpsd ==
  In1 : Inport  OutDataType=sfix(16)  OutScaling=2^0
  lcpsd : M-S-Function  Tag=lcpsd  FunctionName=ltpdasim
  Out1 : Outport  OutDataType=sfix(16)  OutScaling=2^0
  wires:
  In1/1 -> lcpsd/1
  lcpsd/1 -> Out1/1

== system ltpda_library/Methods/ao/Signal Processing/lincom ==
  In1 : Inport  OutDataType=sfix(16)  OutScaling=2^0
  lincom : M-S-Function  Tag=lincom  FunctionName=ltpdasim
  Out1 : Outport  OutDataType=sfix(16)  OutScaling=2^0
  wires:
  In1/1 -> lincom/1
  lincom/1 -> Out1/1

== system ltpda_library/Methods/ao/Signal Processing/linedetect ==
  In1 : Inport  OutDataType=sfix(16)  OutScaling=2^0
  linedetect : M-S-Function  Tag=linedetect  FunctionName=ltpdasim
  Out1 : Outport  OutDataType=sfix(16)  OutScaling=2^0
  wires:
  In1/1 -> linedetect/1
  linedetect/1 -> Out1/1

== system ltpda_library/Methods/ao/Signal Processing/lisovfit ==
  In1 : Inport  OutDataType=sfix(16)  OutScaling=2^0
  lisovfit : M-S-Function  Tag=lisovfit  FunctionName=ltpdasim
  Out1 : Outport  OutDataType=sfix(16)  OutScaling=2^0
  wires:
  In1/1 -> lisovfit/1
  lisovfit/1 -> Out1/1

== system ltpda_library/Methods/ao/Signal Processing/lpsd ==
  In1 : Inport  OutDataType=sfix(16)  OutScaling=2^0
  lpsd : M-S-Function  Tag=lpsd  FunctionName=ltpdasim
  Out1 : Outport  OutDataType=sfix(16)  OutScaling=2^0
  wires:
  In1/1 -> lpsd/1
  lpsd/1 -> Out1/1

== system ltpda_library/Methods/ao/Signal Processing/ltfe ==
  In1 : Inport  OutDataType=sfix(16)  OutScaling=2^0
  ltfe : M-S-Function  Tag=ltfe  FunctionName=ltpdasim
  Out1 : Outport  OutDataType=sfix(16)  OutScaling=2^0
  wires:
  In1/1 -> ltfe/1
  ltfe/1 -> Out1/1

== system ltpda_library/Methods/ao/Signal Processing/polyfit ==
  In1 : Inport  OutDataType=sfix(16)  OutScaling=2^0
  polyfit : M-S-Function  Tag=polyfit  FunctionName=ltpdasim
  Out1 : Outport  OutDataType=sfix(16)  OutScaling=2^0
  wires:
  In1/1 -> polyfit/1
  polyfit/1 -> Out1/1

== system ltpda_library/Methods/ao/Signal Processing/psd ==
  In1 : Inport  OutDataType=sfix(16)  OutScaling=2^0
  psd : M-S-Function  Tag=psd  FunctionName=ltpdasim
  Out1 : Outport  OutDataType=sfix(16)  OutScaling=2^0
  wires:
  In1/1 -> psd/1
  psd/1 -> Out1/1

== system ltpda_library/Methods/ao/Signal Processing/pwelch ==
  In1 : Inport  OutDataType=sfix(16)  OutScaling=2^0
  pwelch : M-S-Function  Tag=pwelch  FunctionName=ltpdasim
  Out1 : Outport  OutDataType=sfix(16)  OutScaling=2^0
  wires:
  In1/1 -> pwelch/1
  pwelch/1 -> Out1/1

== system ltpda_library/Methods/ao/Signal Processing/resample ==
  In1 : Inport  OutDataType=sfix(16)  OutScaling=2^0
  resample : M-S-Function  Tag=resample  FunctionName=ltpdasim
  Out1 : Outport  OutDataType=sfix(16)  OutScaling=2^0
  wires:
  In1/1 -> resample/1
  resample/1 -> Out1/1

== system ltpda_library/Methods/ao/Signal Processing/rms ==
  In1 : Inport  OutDataType=sfix(16)  OutScaling=2^0
  rms : M-S-Function  Tag=rms  FunctionName=ltpdasim
  Out1 : Outport  OutDataType=sfix(16)  OutScaling=2^0
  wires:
  In1/1 -> rms/1
  rms/1 -> Out1/1

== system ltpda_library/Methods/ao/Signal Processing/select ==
  In1 : Inport  OutDataType=sfix(16)  OutScaling=2^0
  select : M-S-Function  Tag=select  FunctionName=ltpdasim
  Out1 : Outport  OutDataType=sfix(16)  OutScaling=2^0
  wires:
  In1/1 -> select/1
  select/1 -> Out1/1

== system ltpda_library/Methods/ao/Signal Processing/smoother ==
  In1 : Inport  OutDataType=sfix(16)  OutScaling=2^0
  smoother : M-S-Function  Tag=smoother  FunctionName=ltpdasim
  Out1 : Outport  OutDataType=sfix(16)  OutScaling=2^0
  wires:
  In1/1 -> smoother/1
  smoother/1 -> Out1/1

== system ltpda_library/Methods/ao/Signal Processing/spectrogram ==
  In1 : Inport  OutDataType=sfix(16)  OutScaling=2^0
  spectrogram : M-S-Function  Tag=spectrogram  FunctionName=ltpdasim
  Out1 : Outport  OutDataType=sfix(16)  OutScaling=2^0
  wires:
  In1/1 -> spectrogram/1
  spectrogram/1 -> Out1/1

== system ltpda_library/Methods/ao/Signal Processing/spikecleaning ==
  In1 : Inport  OutDataType=sfix(16)  OutScaling=2^0
  spikecleaning : M-S-Function  Tag=spikecleaning  FunctionName=ltpdasim
  Out1 : Outport  OutDataType=sfix(16)  OutScaling=2^0
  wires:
  In1/1 -> spikecleaning/1
  spikecleaning/1 -> Out1/1

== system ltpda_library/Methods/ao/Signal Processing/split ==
  In1 : Inport  OutDataType=sfix(16)  OutScaling=2^0
  split : M-S-Function  Tag=split  FunctionName=ltpdasim
  Out1 : Outport  OutDataType=sfix(16)  OutScaling=2^0
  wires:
  In1/1 -> split/1
  split/1 -> Out1/1

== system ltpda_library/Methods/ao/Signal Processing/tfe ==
  In1 : Inport  OutDataType=sfix(16)  OutScaling=2^0
  tfe : M-S-Function  Tag=tfe  FunctionName=ltpdasim
  Out1 : Outport  OutDataType=sfix(16)  OutScaling=2^0
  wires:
  In1/1 -> tfe/1
  tfe/1 -> Out1/1

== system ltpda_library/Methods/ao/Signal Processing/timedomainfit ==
  In1 : Inport  OutDataType=sfix(16)  OutScaling=2^0
  timedomainfit : M-S-Function  Tag=timedomainfit  FunctionName=ltpdasim
  Out1 : Outport  OutDataType=sfix(16)  OutScaling=2^0
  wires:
  In1/1 -> timedomainfit/1
  timedomainfit/1 -> Out1/1

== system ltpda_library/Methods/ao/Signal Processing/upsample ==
  In1 : Inport  OutDataType=sfix(16)  OutScaling=2^0
  upsample : M-S-Function  Tag=upsample  FunctionName=ltpdasim
  Out1 : Outport  OutDataType=sfix(16)  OutScaling=2^0
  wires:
  In1/1 -> upsample/1
  upsample/1 -> Out1/1

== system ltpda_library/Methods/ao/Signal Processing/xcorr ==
  In1 : Inport  OutDataType=sfix(16)  OutScaling=2^0
  xcorr : M-S-Function  Tag=xcorr  FunctionName=ltpdasim
  Out1 : Outport  OutDataType=sfix(16)  OutScaling=2^0
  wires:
  In1/1 -> xcorr/1
  xcorr/1 -> Out1/1

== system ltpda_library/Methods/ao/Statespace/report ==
  In1 : Inport  OutDataType=sfix(16)  OutScaling=2^0
  report : M-S-Function  Tag=report  FunctionName=ltpdasim
  Out1 : Outport  OutDataType=sfix(16)  OutScaling=2^0
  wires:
  In1/1 -> report/1
  report/1 -> Out1/1

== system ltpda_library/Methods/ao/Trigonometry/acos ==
  In1 : Inport  OutDataType=sfix(16)  OutScaling=2^0
  acos : M-S-Function  Tag=acos  FunctionName=ltpdasim
  Out1 : Outport  OutDataType=sfix(16)  OutScaling=2^0
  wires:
  In1/1 -> acos/1
  acos/1 -> Out1/1

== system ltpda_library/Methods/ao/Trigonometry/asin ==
  In1 : Inport  OutDataType=sfix(16)  OutScaling=2^0
  asin : M-S-Function  Tag=asin  FunctionName=ltpdasim
  Out1 : Outport  OutDataType=sfix(16)  OutScaling=2^0
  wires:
  In1/1 -> asin/1
  asin/1 -> Out1/1

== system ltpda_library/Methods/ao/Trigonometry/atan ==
  In1 : Inport  OutDataType=sfix(16)  OutScaling=2^0
  atan : M-S-Function  Tag=atan  FunctionName=ltpdasim
  Out1 : Outport  OutDataType=sfix(16)  OutScaling=2^0
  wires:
  In1/1 -> atan/1
  atan/1 -> Out1/1

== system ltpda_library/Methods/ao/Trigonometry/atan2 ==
  In1 : Inport  OutDataType=sfix(16)  OutScaling=2^0
  atan2 : M-S-Function  Tag=atan2  FunctionName=ltpdasim
  Out1 : Outport  OutDataType=sfix(16)  OutScaling=2^0
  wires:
  In1/1 -> atan2/1
  atan2/1 -> Out1/1

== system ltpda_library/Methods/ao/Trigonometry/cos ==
  In1 : Inport  OutDataType=sfix(16)  OutScaling=2^0
  cos : M-S-Function  Tag=cos  FunctionName=ltpdasim
  Out1 : Outport  OutDataType=sfix(16)  OutScaling=2^0
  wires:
  In1/1 -> cos/1
  cos/1 -> Out1/1

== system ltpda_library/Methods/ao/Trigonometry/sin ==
  In1 : Inport  OutDataType=sfix(16)  OutScaling=2^0
  sin : M-S-Function  Tag=sin  FunctionName=ltpdasim
  Out1 : Outport  OutDataType=sfix(16)  OutScaling=2^0
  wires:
  In1/1 -> sin/1
  sin/1 -> Out1/1

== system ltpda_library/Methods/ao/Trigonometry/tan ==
  In1 : Inport  OutDataType=sfix(16)  OutScaling=2^0
  tan : M-S-Function  Tag=tan  FunctionName=ltpdasim
  Out1 : Outport  OutDataType=sfix(16)  OutScaling=2^0
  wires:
  In1/1 -> tan/1
  tan/1 -> Out1/1

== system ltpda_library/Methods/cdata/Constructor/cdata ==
  Ground : Ground
  cdata : M-S-Function  Tag=cdata  FunctionName=ltpdasim
  Out1 : Outport  OutDataType=sfix(16)  OutScaling=2^0
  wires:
  Ground/1 -> cdata/1
  cdata/1 -> Out1/1

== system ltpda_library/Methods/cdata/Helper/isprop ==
  In1 : Inport  OutDataType=sfix(16)  OutScaling=2^0
  isprop : M-S-Function  Tag=isprop  FunctionName=ltpdasim
  Out1 : Outport  OutDataType=sfix(16)  OutScaling=2^0
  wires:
  In1/1 -> isprop/1
  isprop/1 -> Out1/1

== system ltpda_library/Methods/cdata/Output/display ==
  In1 : Inport  OutDataType=sfix(16)  OutScaling=2^0
  Terminator : Terminator
  display : M-S-Function  Tag=display  FunctionName=ltpdasim
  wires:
  display/1 -> Terminator/1
  In1/1 -> display/1

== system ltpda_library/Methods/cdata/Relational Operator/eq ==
  In1 : Inport  OutDataType=sfix(16)  OutScaling=2^0
  eq : M-S-Function  Tag=eq  FunctionName=ltpdasim
  Out1 : Outport  OutDataType=sfix(16)  OutScaling=2^0
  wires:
  In1/1 -> eq/1
  eq/1 -> Out1/1

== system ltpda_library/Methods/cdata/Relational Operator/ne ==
  In1 : Inport  OutDataType=sfix(16)  OutScaling=2^0
  ne : M-S-Function  Tag=ne  FunctionName=ltpdasim
  Out1 : Outport  OutDataType=sfix(16)  OutScaling=2^0
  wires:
  In1/1 -> ne/1
  ne/1 -> Out1/1

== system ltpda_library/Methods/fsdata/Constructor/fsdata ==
  Ground : Ground
  fsdata : M-S-Function  Tag=fsdata  FunctionName=ltpdasim
  Out1 : Outport  OutDataType=sfix(16)  OutScaling=2^0
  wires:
  Ground/1 -> fsdata/1
  fsdata/1 -> Out1/1

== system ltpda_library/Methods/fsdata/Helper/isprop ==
  In1 : Inport  OutDataType=sfix(16)  OutScaling=2^0
  isprop : M-S-Function  Tag=isprop  FunctionName=ltpdasim
  Out1 : Outport  OutDataType=sfix(16)  OutScaling=2^0
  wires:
  In1/1 -> isprop/1
  isprop/1 -> Out1/1

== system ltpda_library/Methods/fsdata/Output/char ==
  In1 : Inport  OutDataType=sfix(16)  OutScaling=2^0
  Terminator : Terminator
  char : M-S-Function  Tag=char  FunctionName=ltpdasim
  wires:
  char/1 -> Terminator/1
  In1/1 -> char/1

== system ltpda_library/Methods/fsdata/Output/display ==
  In1 : Inport  OutDataType=sfix(16)  OutScaling=2^0
  Terminator : Terminator
  display : M-S-Function  Tag=display  FunctionName=ltpdasim
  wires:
  display/1 -> Terminator/1
  In1/1 -> display/1

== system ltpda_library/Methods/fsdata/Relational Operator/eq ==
  In1 : Inport  OutDataType=sfix(16)  OutScaling=2^0
  eq : M-S-Function  Tag=eq  FunctionName=ltpdasim
  Out1 : Outport  OutDataType=sfix(16)  OutScaling=2^0
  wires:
  In1/1 -> eq/1
  eq/1 -> Out1/1

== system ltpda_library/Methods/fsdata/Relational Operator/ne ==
  In1 : Inport  OutDataType=sfix(16)  OutScaling=2^0
  ne : M-S-Function  Tag=ne  FunctionName=ltpdasim
  Out1 : Outport  OutDataType=sfix(16)  OutScaling=2^0
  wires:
  In1/1 -> ne/1
  ne/1 -> Out1/1

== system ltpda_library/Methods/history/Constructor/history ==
  Ground : Ground
  history : M-S-Function  Tag=history  FunctionName=ltpdasim
  Out1 : Outport  OutDataType=sfix(16)  OutScaling=2^0
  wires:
  Ground/1 -> history/1
  history/1 -> Out1/1

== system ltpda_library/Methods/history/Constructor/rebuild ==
  Ground : Ground
  rebuild : M-S-Function  Tag=rebuild  FunctionName=ltpdasim
  Out1 : Outport  OutDataType=sfix(16)  OutScaling=2^0
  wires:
  Ground/1 -> rebuild/1
  rebuild/1 -> Out1/1

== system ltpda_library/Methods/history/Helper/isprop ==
  In1 : Inport  OutDataType=sfix(16)  OutScaling=2^0
  isprop : M-S-Function  Tag=isprop  FunctionName=ltpdasim
  Out1 : Outport  OutDataType=sfix(16)  OutScaling=2^0
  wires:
  In1/1 -> isprop/1
  isprop/1 -> Out1/1

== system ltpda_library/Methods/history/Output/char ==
  In1 : Inport  OutDataType=sfix(16)  OutScaling=2^0
  Terminator : Terminator
  char : M-S-Function  Tag=char  FunctionName=ltpdasim
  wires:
  char/1 -> Terminator/1
  In1/1 -> char/1

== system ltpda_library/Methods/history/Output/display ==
  In1 : Inport  OutDataType=sfix(16)  OutScaling=2^0
  Terminator : Terminator
  display : M-S-Function  Tag=display  FunctionName=ltpdasim
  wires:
  display/1 -> Terminator/1
  In1/1 -> display/1

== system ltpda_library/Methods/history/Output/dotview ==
  In1 : Inport  OutDataType=sfix(16)  OutScaling=2^0
  Terminator : Terminator
  dotview : M-S-Function  Tag=dotview  FunctionName=ltpdasim
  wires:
  dotview/1 -> Terminator/1
  In1/1 -> dotview/1

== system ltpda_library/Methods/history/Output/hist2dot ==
  In1 : Inport  OutDataType=sfix(16)  OutScaling=2^0
  Terminator : Terminator
  hist2dot : M-S-Function  Tag=hist2dot  FunctionName=ltpdasim
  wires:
  hist2dot/1 -> Terminator/1
  In1/1 -> hist2dot/1

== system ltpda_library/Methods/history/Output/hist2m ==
  In1 : Inport  OutDataType=sfix(16)  OutScaling=2^0
  Terminator : Terminator
  hist2m : M-S-Function  Tag=hist2m  FunctionName=ltpdasim
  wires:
  hist2m/1 -> Terminator/1
  In1/1 -> hist2m/1

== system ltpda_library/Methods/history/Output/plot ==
  In1 : Inport  OutDataType=sfix(16)  OutScaling=2^0
  Terminator : Terminator
  plot : M-S-Function  Tag=plot  FunctionName=ltpdasim
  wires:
  plot/1 -> Terminator/1
  In1/1 -> plot/1

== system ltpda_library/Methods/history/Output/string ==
  In1 : Inport  OutDataType=sfix(16)  OutScaling=2^0
  Terminator : Terminator
  string : M-S-Function  Tag=string  FunctionName=ltpdasim
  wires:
  string/1 -> Terminator/1
  In1/1 -> string/1

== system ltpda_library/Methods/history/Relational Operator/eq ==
  In1 : Inport  OutDataType=sfix(16)  OutScaling=2^0
  eq : M-S-Function  Tag=eq  FunctionName=ltpdasim
  Out1 : Outport  OutDataType=sfix(16)  OutScaling=2^0
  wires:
  In1/1 -> eq/1
  eq/1 -> Out1/1

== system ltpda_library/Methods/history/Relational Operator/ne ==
  In1 : Inport  OutDataType=sfix(16)  OutScaling=2^0
  ne : M-S-Function  Tag=ne  FunctionName=ltpdasim
  Out1 : Outport  OutDataType=sfix(16)  OutScaling=2^0
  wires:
  In1/1 -> ne/1
  ne/1 -> Out1/1

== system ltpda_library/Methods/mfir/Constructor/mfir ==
  Ground : Ground
  mfir : M-S-Function  Tag=mfir  FunctionName=ltpdasim
  Out1 : Outport  OutDataType=sfix(16)  OutScaling=2^0
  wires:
  Ground/1 -> mfir/1
  mfir/1 -> Out1/1

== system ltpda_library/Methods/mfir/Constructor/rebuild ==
  Ground : Ground
  rebuild : M-S-Function  Tag=rebuild  FunctionName=ltpdasim
  Out1 : Outport  OutDataType=sfix(16)  OutScaling=2^0
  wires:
  Ground/1 -> rebuild/1
  rebuild/1 -> Out1/1

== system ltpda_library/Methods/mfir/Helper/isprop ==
  In1 : Inport  OutDataType=sfix(16)  OutScaling=2^0
  isprop : M-S-Function  Tag=isprop  FunctionName=ltpdasim
  Out1 : Outport  OutDataType=sfix(16)  OutScaling=2^0
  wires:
  In1/1 -> isprop/1
  isprop/1 -> Out1/1

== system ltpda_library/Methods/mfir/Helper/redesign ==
  In1 : Inport  OutDataType=sfix(16)  OutScaling=2^0
  redesign : M-S-Function  Tag=redesign  FunctionName=ltpdasim
  Out1 : Outport  OutDataType=sfix(16)  OutScaling=2^0
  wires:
  In1/1 -> redesign/1
  redesign/1 -> Out1/1

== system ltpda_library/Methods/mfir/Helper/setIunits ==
  In1 : Inport  OutDataType=sfix(16)  OutScaling=2^0
  setIunits : M-S-Function  Tag=setIunits  FunctionName=ltpdasim
  Out1 : Outport  OutDataType=sfix(16)  OutScaling=2^0
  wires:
  In1/1 -> setIunits/1
  setIunits/1 -> Out1/1

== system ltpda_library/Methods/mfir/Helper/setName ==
  In1 : Inport  OutDataType=sfix(16)  OutScaling=2^0
  setName : M-S-Function  Tag=setName  FunctionName=ltpdasim
  Out1 : Outport  OutDataType=sfix(16)  OutScaling=2^0
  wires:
  In1/1 -> setName/1
  setName/1 -> Out1/1

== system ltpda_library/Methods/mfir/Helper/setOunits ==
  In1 : Inport  OutDataType=sfix(16)  OutScaling=2^0
  setOunits : M-S-Function  Tag=setOunits  FunctionName=ltpdasim
  Out1 : Outport  OutDataType=sfix(16)  OutScaling=2^0
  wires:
  In1/1 -> setOunits/1
  setOunits/1 -> Out1/1

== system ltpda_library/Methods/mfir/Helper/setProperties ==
  In1 : Inport  OutDataType=sfix(16)  OutScaling=2^0
  setProperties : M-S-Function  Tag=setProperties  FunctionName=ltpdasim
  Out1 : Outport  OutDataType=sfix(16)  OutScaling=2^0
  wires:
  In1/1 -> setProperties/1
  setProperties/1 -> Out1/1

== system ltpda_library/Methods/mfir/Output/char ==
  In1 : Inport  OutDataType=sfix(16)  OutScaling=2^0
  Terminator : Terminator
  char : M-S-Function  Tag=char  FunctionName=ltpdasim
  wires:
  char/1 -> Terminator/1
  In1/1 -> char/1

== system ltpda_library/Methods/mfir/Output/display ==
  In1 : Inport  OutDataType=sfix(16)  OutScaling=2^0
  Terminator : Terminator
  display : M-S-Function  Tag=display  FunctionName=ltpdasim
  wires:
  display/1 -> Terminator/1
  In1/1 -> display/1
